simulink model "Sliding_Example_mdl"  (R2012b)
settings: Solver=ode45  SolverMode=SingleTasking  StartTime=0.0  StopTime=4.0  RelTol=1e-6  AbsTol=1e-6
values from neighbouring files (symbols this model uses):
  a0 = 1    [Sliding_Example.m]
  a1 = 2    [Sliding_Example.m]
  alpha = 3    [Sliding_Example.m]
  c1 = 1.5    [Sliding_Example.m]
  Tc = Tfin/4000    (= 0.001)    [Sliding_Example.m]
  x1_0 = In_Con(jj,1)    [Sliding_Example.m]
  x2_0 = In_Con(jj,2)    [Sliding_Example.m]
undefined symbols (not defined in the file or in its folder): sgn

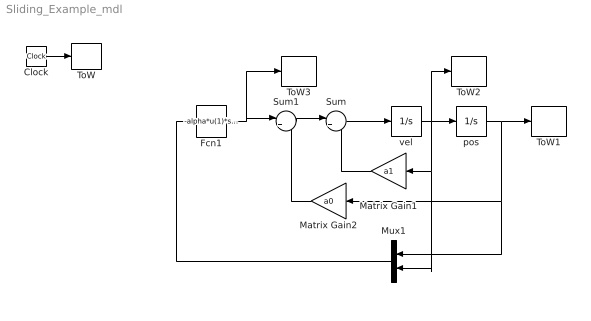
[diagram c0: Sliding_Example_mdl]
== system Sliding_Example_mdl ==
  Clock : Clock
  Fcn1 : Fcn  Expr=-alpha*u(1)*sgn(u(1)*(c1*u(1)+u(2)))  SampleTime=Tc
  Matrix Gain1 : Gain  Gain=a1
  Matrix Gain2 : Gain  Gain=a0
  Mux1 : Mux  Inputs=2
  Sum : Sum  Inputs=|+-
  Sum1 : Sum  Inputs=|+-
  ToW : ToWorkspace  VariableName=t  SampleTime=Tc
  ToW1 : ToWorkspace  VariableName=x1  SampleTime=Tc
  ToW2 : ToWorkspace  VariableName=x2  SampleTime=Tc
  ToW3 : ToWorkspace  VariableName=u  SampleTime=Tc
  pos : Integrator  InitialCondition=x1_0
  vel : Integrator  InitialCondition=x2_0
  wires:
  vel/1 -> pos/1, ToW2/1, Matrix Gain1/1, Mux1/2
  Clock/1 -> ToW/1
  pos/1 -> ToW1/1, Matrix Gain2/1, Mux1/1
  Matrix Gain1/1 -> Sum/2
  Sum1/1 -> Sum/1
  Sum/1 -> vel/1
  Matrix Gain2/1 -> Sum1/2
  Mux1/1 -> Fcn1/1
  Fcn1/1 -> Sum1/1, ToW3/1
